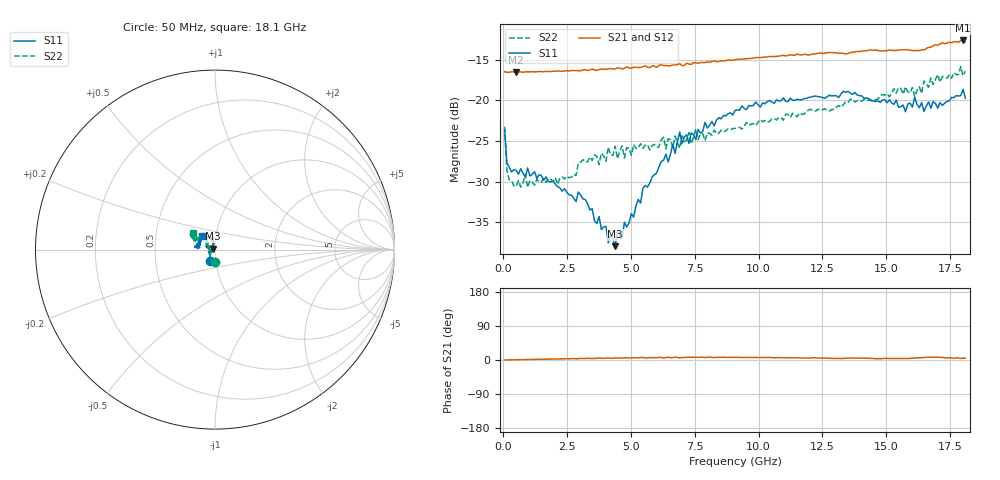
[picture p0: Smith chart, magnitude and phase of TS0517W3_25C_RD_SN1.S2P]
! Network Analyzer HP8720D.06.14 Serial No. US36140669
! 17 Jun 2005  08:59:24
! Frequency  S11  S21  S12  S22
# HZ  S  DB R 50
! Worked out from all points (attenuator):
!   201 points, 50 MHz to 18.1 GHz, reference 50 ohm
!   highest |S21| = -12.63 dB at 18.01 GHz (marker M1); lowest = -16.6 dB at 501.2 MHz (marker M2)
!   lowest |S11| = -37.9 dB at 4.382 GHz (marker M3), VSWR 1.03, Z = 48.9 + j0.557 ohm
!   |S11| at or under -10 dB: start of sweep to end of sweep
!   |S22| runs from -30.7 to -15.8 dB; largest |S21 - S12| = 0.0061
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5e7  -23.61 -112.5  -16.47 0.1  -16.48 0.2  -23.25 -89.1
1.4025e8  -27.71 -134.6  -16.55 0.2  -16.55 0.2  -28.64 -128.3
5.0125e8  -28.61 -154.8  -16.55 0.6  -16.53 0.6  -30.61 -166.7
8.6225e8  -29.45 -163.5  -16.49 1.2  -16.52 1.4  -29.10 -173.9
9.525e8  -28.31 -160.0  -16.49 1.7  -16.50 1.4  -30.70 -177.7
2.12575e9  -30.62 -156.9  -16.38 2.6  -16.41 2.7  -30.35 159.6
3.1185e9  -32.12 -160.3  -16.25 3.9  -16.30 3.8  -27.30 165.1
3.75025e9  -34.28 -171.7  -16.20 5.2  -16.25 5.2  -27.89 160.6
4.382e9  -37.94 153.3  -16.14 5.6  -16.09 5.0  -25.66 159.3
4.47225e9  -36.01 142.5  -16.01 5.4  -16.06 5.7  -27.18 162.3
4.65275e9  -36.98 132.0  -16.16 5.3  -16.04 5.5  -25.60 161.8
4.743e9  -34.98 133.4  -16.05 5.7  -16.08 5.7  -27.09 157.1
6.09675e9  -28.17 102.8  -15.70 6.7  -15.65 6.5  -25.72 149.5
6.7285e9  -26.54 106.9  -15.65 7.7  -15.74 7.0  -24.39 143.5
6.909e9  -23.89 105.9  -15.47 5.7  -15.60 6.2  -25.88 137.8
7.27e9  -25.30 102.6  -15.54 7.5  -15.55 6.6  -23.96 140.0
9.075e9  -21.25 124.7  -15.00 7.0  -14.99 7.0  -23.45 131.5
1.21435e10  -19.50 163.0  -14.30 6.1  -14.29 5.9  -21.26 133.7
1.512175e10  -19.93 171.8  -13.80 4.1  -13.78 4.4  -19.57 149.4
1.64755e10  -21.36 163.8  -13.79 6.9  -13.74 7.3  -17.63 150.5
1.800975e10  -18.64 132.9  -12.63 4.9  -12.74 5.0  -16.97 149.8
1.81e10  -19.73 134.5  -12.82 4.9  -12.85 3.6  -16.41 143.0
